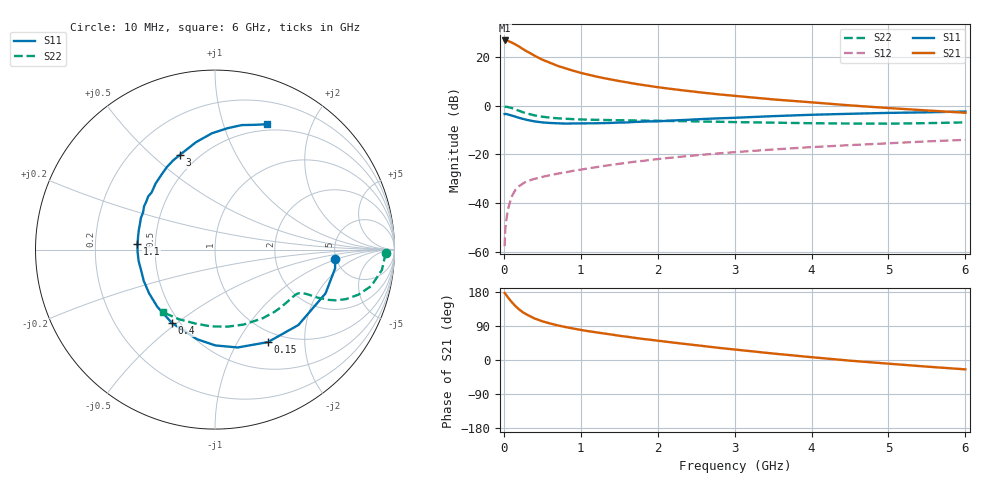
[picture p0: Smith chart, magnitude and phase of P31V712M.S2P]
! SIEMENS Small Signal Semiconductors
! BFP181
! Si NPN RF Bipolar Junction Transistor in SOT143
! VCE = 1.75 V  IC = 12 mA
! Common Emitter S-Parameters:  March  1996
# GHz  S  MA  R  50
!  f  S11  S21  S12  S22
! GHz  MAG  ANG  MAG  ANG  MAG  ANG  MAG  ANG
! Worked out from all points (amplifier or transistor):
!   36 points, 10 MHz to 6 GHz, reference 50 ohm
!   highest |S21| = 26.8 dB at 10 MHz (marker M1)
!   |S21| within 3 dB of that: start of sweep to 222.2 MHz
!   unconditionally stable (mu >= 1): 678.3 MHz to end of sweep
!   at 250 MHz: K = 0.49, MSG = 27.6 dB, |S12| = -32.0 dB
!   at 1.4 GHz: K = 1.32, MAG = 14.1 dB, |S12| = -24.3 dB
!   at 6 GHz: K = 1.09, MAG = 3.7 dB, |S12| = -14.1 dB
!   S11 on the Smith chart (normalised r, x): 10 MHz: 4.89, -0.93; 150 MHz: 0.85, -1.35; 400 MHz: 0.45, -0.48; 1.1 GHz: 0.40, +0.03; 3 GHz: 0.40, +0.62; 6 GHz: 0.43, +1.41
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0.01  0.6706 -4.5  21.79 177.2  0.0013 86.9  0.9519 -1.1
0.02  0.6774 -8.9  21.78 174.8  0.0031 83.5  0.9466 -2.6
0.05  0.6624 -21.6  21.42 166.1  0.0071 81.9  0.9371 -6.9
0.1  0.6264 -42.1  19.85 153.5  0.0134 70.7  0.8941 -13.1
0.15  0.5939 -60.2  18.08 142.4  0.0186 63.6  0.8365 -17.5
0.2  0.5598 -76.9  16.26 133.2  0.0223 59.0  0.7804 -20.7
0.25  0.5339 -89.8  14.43 125.6  0.0252 54.9  0.7299 -22.8
0.3  0.5092 -101.4  13 119.8  0.0281 53.1  0.691 -23.9
0.4  0.4741 -120.5  10.59 109.6  0.0314 50.0  0.631 -25.1
0.5  0.4525 -135.3  8.789 102.2  0.0344 48.4  0.5923 -25.5
0.6  0.4406 -146.5  7.589 96.5  0.0373 48.4  0.5665 -25.9
0.7  0.4335 -156.2  6.55 91.4  0.0401 48.6  0.5494 -26.3
0.9  0.4304 -171.7  5.22 83.2  0.0458 49.2  0.528 -27.4
1.1  0.4331 175.6  4.314 76.0  0.0518 50.7  0.5152 -29.1
1.5  0.4489 156.9  3.198 64.0  0.0639 50.8  0.5008 -33.8
1.8  0.4677 144.8  2.663 55.8  0.0731 50.7  0.4926 -38.0
2.2  0.4953 131.9  2.176 46.0  0.086 49.0  0.4825 -44.3
3  0.5625 110.4  1.587 27.7  0.1107 44.3  0.4584 -58.7
3.5  0.608 100.0  1.343 17.1  0.1257 40.9  0.4471 -69.1
4.5  0.6799 84.1  1.012 -1.8  0.1544 33.2  0.4287 -92.7
5.5  0.7285 72.6  0.796 -17.5  0.1843 25.7  0.4367 -117.3
6  0.757 67.3  0.713 -24.7  0.1983 21.4  0.4528 -129.4
